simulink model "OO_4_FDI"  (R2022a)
settings: Solver=VariableStepAuto  StartTime=0.0  StopTime=300  RelTol=1e-3
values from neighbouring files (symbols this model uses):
  Ao1 = Am - Ko1*Cm(1,:)    [OO_design.m]
  Ao2 = Am - Ko2*Cm(2,:)    [OO_design.m]
  Bo1 = [Bm Ko1]    [OO_design.m]
  Bo2 = [Bm Ko2]    [OO_design.m]
  C = 6.3000e-04    (= 0.00063)    [maglev_init.m]
  Co1 = Cm(1,:)    [OO_design.m]
  Co2 = Cm(2,:)    [OO_design.m]
  Do1 = zeros(1,2)    [OO_design.m]
  Do2 = zeros(1,2)    [OO_design.m]
  g = 9.80    (= 9.8)    [maglev_init.m]
  K = 1.0e+03 * [-2.4567   -0.1235    0.0237]    [maglev_init.m]
  L1 = 0.6000    (= 0.6)    [maglev_init.m]
  m = 0.0300    (= 0.03)    [maglev_init.m]
  mpert = 0    [maglev_init.m]
  R = 45    [maglev_init.m]
  Ts = 0.005    [maglev_init.m]    (also in train_net.m)
  x1_0 = 0.1    [maglev_init.m]
  x1_d = 0.05    [maglev_init.m]
  x2_0 = 0    [maglev_init.m]
  x2_d = 0    [maglev_init.m]
  x3_0 = 0.2    [maglev_init.m]

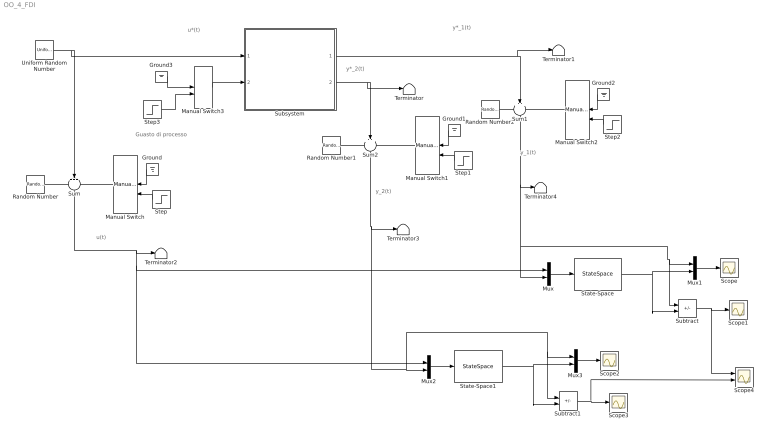
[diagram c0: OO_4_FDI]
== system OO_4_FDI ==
  note: y_2(t)
  note: y*_1(t)
  note: u(t)
  note: y*_2(t)
  note: y_1(t)
  note: u*(t)
  note: Guasto di processo
  Ground{,1..3} (4 alike) : Ground
  Manual Switch{,1..3} (4 alike) : ManualSwitch
  Mux{,1..3} (4 alike) : Mux  Inputs=2
  Random Number : RandomNumber  Variance=1e-9  Seed=1  SampleTime=Ts
  Random Number1 : RandomNumber  Variance=1e-6  Seed=3  SampleTime=Ts
  Random Number2 : RandomNumber  Variance=1e-9  Seed=2  SampleTime=Ts
  Scope{,1..3} (4 alike) : Scope
  Scope4 : Scope  NumInputPorts=2
  State-Space : StateSpace  A=Ao1  B=Bo1  C=Co1  D=Do1  InitialCondition=0
  State-Space1 : StateSpace  A=Ao2  B=Bo2  C=Co2  D=Do2  InitialCondition=0
  Step : Step  Time=150  SampleTime=0
  Step1 : Step  Time=150  SampleTime=0
  Step2 : Step  Time=150  SampleTime=0
  Step3 : Step  Time=150  After=2*R  SampleTime=0
  Subsystem : Subsystem
  Subtract : Sum  Inputs=+-
  Subtract1 : Sum  Inputs=+-
  Sum : Sum  Inputs=+++
  Sum1 : Sum  Inputs=+++
  Sum2 : Sum  Inputs=+++
  Terminator{,1..4} (5 alike) : Terminator
  Uniform Random Number : UniformRandomNumber  Minimum=x1_d*0.9  Maximum=x1_d*1.1  Seed=1  SampleTime=0.5
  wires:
  Subsystem/1(Out1) -> Terminator1/1, Sum1/2
  Subsystem/2(Out2) -> Terminator/1, Sum2/2
  Random Number/1 -> Sum/1
  Manual Switch/1 -> Sum/3
  Manual Switch2/1 -> Sum1/3
  Manual Switch1/1 -> Sum2/3
  Random Number1/1 -> Sum2/1
  Ground/1 -> Manual Switch/1
  Step/1 -> Manual Switch/2
  Ground1/1 -> Manual Switch1/1
  Step1/1 -> Manual Switch1/2
  Sum2/1 -> Mux3/1, Subtract1/1, Mux2/2, Terminator3/1
  Random Number2/1 -> Sum1/1
  Ground2/1 -> Manual Switch2/1
  Step2/1 -> Manual Switch2/2
  Sum1/1 -> Subtract/1, Mux1/1, Mux/2, Terminator4/1
  Manual Switch3/1 -> Subsystem/2(fs)
  Ground3/1 -> Manual Switch3/1
  Uniform Random Number/1 -> Subsystem/1(u), Sum/2
  Step3/1 -> Manual Switch3/2
  Sum/1 -> Mux2/1, Mux/1, Terminator2/1
  Mux/1 -> State-Space/1
  State-Space/1 -> Subtract/2, Mux1/2
  Mux1/1 -> Scope/1
  Subtract/1 -> Scope4/1, Scope1/1
  State-Space1/1 -> Subtract1/2, Mux3/2
  Subtract1/1 -> Scope4/2, Scope3/1
  Mux2/1 -> State-Space1/1
  Mux3/1 -> Scope2/1

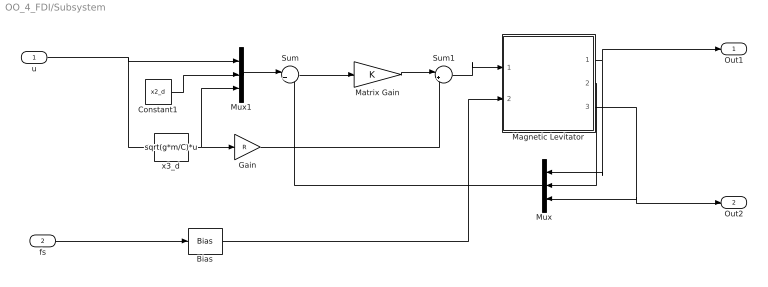
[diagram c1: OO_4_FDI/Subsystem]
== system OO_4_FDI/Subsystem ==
  u : Inport
  fs : Inport  Port=2
  Bias : Bias  Bias=R
  Constant1 : Constant  Value=x2_d
  Gain : Gain  Gain=R
  Magnetic Levitator : Subsystem  mask{m=m+mpert, R=R, L1=L1, C=C, g=g}
      mask prompts: m "ball's mass (m)"; R "Electromagnet's resistance (R)"; L1 "Electromagnet's inductance (L1)"; C "Magnetic force constant (C)"; g "Gravitational acceleration (g)"
  Matrix Gain : Gain  Gain=K  Multiplication=Matrix(K*u)  SaturateOnIntegerOverflow=on
  Mux : Mux  Inputs=3
  Mux1 : Mux  Inputs=3
  Sum : Sum  Inputs=|+-  InputSameDT=on  SaturateOnIntegerOverflow=on
  Sum1 : Sum  Inputs=|++  InputSameDT=on  SaturateOnIntegerOverflow=on
  x3_d : Fcn  Expr=sqrt(g*m/C)*u
  Out1 : Outport
  Out2 : Outport  Port=2
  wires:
  u/1 -> x3_d/1, Mux1/1
  Magnetic Levitator/2(x2) -> Mux/2
  x3_d/1 -> Mux1/3, Gain/1
  Mux1/1 -> Sum/1
  Gain/1 -> Sum1/2
  Mux/1 -> Sum/2
  Constant1/1 -> Mux1/2
  Sum/1 -> Matrix Gain/1
  Sum1/1 -> Magnetic Levitator/1(u)
  Magnetic Levitator/1(x1) -> Out1/1, Mux/1
  Magnetic Levitator/3(x3) -> Out2/1, Mux/3
  Matrix Gain/1 -> Sum1/1
  Bias/1 -> Magnetic Levitator/2(fs)
  fs/1 -> Bias/1

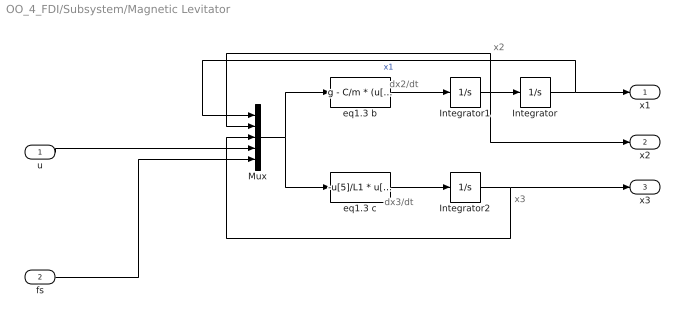
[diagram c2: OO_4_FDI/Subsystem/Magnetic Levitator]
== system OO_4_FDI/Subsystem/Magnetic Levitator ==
  note: x2
  note: x3
  note: dx2/dt
  note: dx3/dt
  u : Inport
  fs : Inport  Port=2
  Integrator : Integrator  InitialCondition=x1_0
  Integrator1 : Integrator  InitialCondition=x2_0
  Integrator2 : Integrator  InitialCondition=x3_0
  Mux : Mux  Inputs=5
  eq1.3 b : Fcn  Expr=g - C/m * (u[3] / u[1])^2
  eq1.3 c : Fcn  Expr=-u[5]/L1 * u[3] + (2*C)/L1 * ( u[2] * u[3] / u[1]^2 ) + 1/L1 * u[4]
  x1 : Outport
  x2 : Outport  Port=2
  x3 : Outport  Port=3
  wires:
  eq1.3 b/1 -> Integrator1/1
  Integrator1/1 -> Integrator/1, Mux/2, x2/1
  eq1.3 c/1 -> Integrator2/1
  Mux/1 -> eq1.3 b/1, eq1.3 c/1
  Integrator/1 -> Mux/1, x1/1  "x1"
  Integrator2/1 -> Mux/3, x3/1
  u/1 -> Mux/4
  fs/1 -> Mux/5
